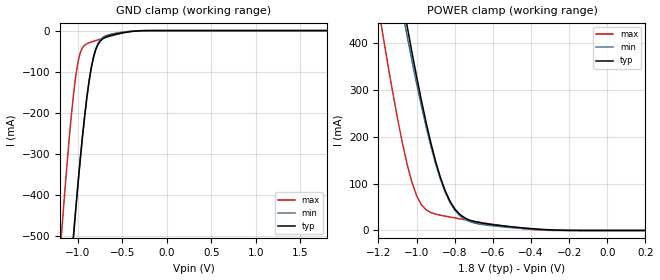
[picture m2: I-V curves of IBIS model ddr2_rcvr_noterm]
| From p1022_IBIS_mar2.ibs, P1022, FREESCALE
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| * P1022 DDR2 Receiver Model - No Termination   *
[Model]   ddr2_rcvr_noterm
Model_type Input
Polarity   Non-Inverting
Vinl = 0.7V
Vinh = 1.1V
|   typ   min   max
C_comp   3.628490e-12   2.023010e-12   4.796400e-12
|   typ   min   max
[Voltage range]   1.8V   1.7V   1.9V
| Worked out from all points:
|   GND clamp passes 1 mA (typ) near -0.33 V on its own axis
|   POWER clamp passes 1 mA (typ) near -0.28 V on its own axis
[GND_clamp]
| Voltage   I(typ)   I(min)   I(max)
-1.8V     -2.78A     -2.734A    -2.433A
-1.2V     -918.5mA   -909.4mA   -538.8mA
-1.175V   -846mA     -838.3mA   -467.5mA
-1.1V     -634.6mA   -630.8mA   -267.7mA
-1.05V    -500.5mA   -498.8mA   -155.7mA
-975mV    -315.3mA   -316.1mA   -54.58mA
-900mV    -162.7mA   -164.1mA   -32.05mA
-850mV    -90.19mA   -90.35mA   -27.79mA
-800mV    -46.39mA   -44.74mA   -24.31mA
-650mV    -12.83mA   -9.896mA   -14.51mA
-300mV    -558.6uA   -261.1uA   -231.9uA
1.8V      1.714uA    9.547uA    12.36nA
[POWER_clamp]
| Voltage   I(typ)   I(min)   I(max)
-1.8V     2.412A     2.266A     2.142A
-1.2V     797.2mA    753.3mA    475mA
-1.175V   734.5mA    694.6mA    412.6mA
-1.1V     552mA      523.4mA    238.4mA
-1.05V    436.4mA    415mA      141.5mA
-1V       328.1mA    313.2mA    74.16mA
-925mV    186.2mA    179.4mA    38.2mA
-875mV    112.7mA    109.2mA    32.53mA
-825mV    62.3mA     59.8mA     28.63mA
-725mV    22.56mA    19.44mA    21.45mA
-350mV    2.574mA    1.808mA    967.2uA
200mV     0A         0A         0A
